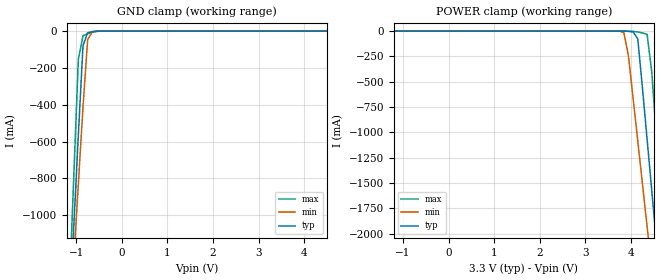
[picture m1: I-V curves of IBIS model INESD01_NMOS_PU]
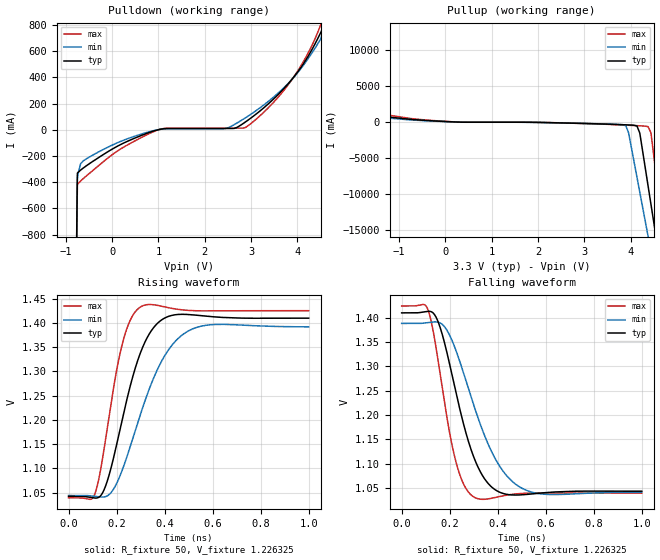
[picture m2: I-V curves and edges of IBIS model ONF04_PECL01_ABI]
|   This file is an IBIS representation of the   |
|   Integrated Device Technology Inc   |
|   ICS844201I-45   |
|   FEMTOCLOCKS CRYSTAL-TO-LVDS CLOCK GENERATOR   |
[IBIS Ver]   4.1
[File name]   844201i_45_3v3.ibs
[File Rev]   1.0
[Date]   3 Mar 2010
[Source]   Originated at Integrated Device Technology, Inc.
[Disclaimer]
IDT hereby grants the user of this IBIS model a non-exclusive,
nontransferable license to use this IBIS model under the following terms.
Before using this IBIS model, the user should read this license.
If the user does not accept these terms,  the IBIS model should be
returned to IDT within 30 days.
   The user is granted this license only to use the IBIS model and
is not granted rights to sell, load, rent, lease or license the IBIS
model in whole or in part, or in modified form to anyone other than
user. User may modify the IBIS model to suit its specific
applications but rights to derivative works and such modifications
shall belong to IDT.
   This IBIS model is provided on an "AS IS" basis and IDT makes
absolutely no warranty with respect to the information contained
herein. IDT DISCLAIMS AND CUSTOMER WAIVES ALL WARRANTIES, EXPRESS
OR IMPLIED, INCLUDING WARRANTIES OF MERCHANTABILITY OR FITNESS FOR
A PARTICULAR PURPOSE. The entire risk as to quality and performance
is with the Customer. ACCORDINGLY, IN NO EVENT SHALL THE COMPANY BE
LIABLE FOR ANY DAMAGES, WHETHER IN CONTRACT OR TORT,INCLUDING ANY
LOST PROFITS OR OTHER INCIDENTAL, CONSEQUENTIAL, EXEMPLARY, OR
PUNITIVE DAMAGES ARISING OUT OF THE USE OR APPLICATION OF THE IBIS
model provided in this package. Further, IDT reserves the right to
make changes without notice to any product herein to improve
reliability, function, or design. IDT does not convey any license
under patent rights or any other intellectual property rights,
including those of third parties.
   IDT is not obligated to provide maintenance or support
for the licensed IBIS model.
[Copyright]   Copyright 2010 by IDT Inc.
[Component]   ICS844201KI-45
[Manufacturer] Integrated Device Technology, Inc.
[Package]
|QFN 16
|lead + wire   typ   min   max
R_pkg   72.4655m   58.886m   86.045m
L_pkg   1.47175nH   1.11650nH   1.77850n
C_pkg   0.07747pF   0.07444pF   0.08050pF
[Pin] signal_name  model_name   R_pin   L_pin   C_pin
1   NC   NC   86.045m   1.77850nH   0.08050pF
2   XTAL_IN   NC   58.886m   1.11650nH   0.07444pF
3   XTAL_OUT  NC   58.886m   1.11650nH   0.07444pF
4   FSEL   INESD01_NMOS_PU   86.045m   1.77850nH   0.08050pF
5   GND   GND   86.045m   1.77850nH   0.08050pF
6   NC   NC   58.886m   1.11650nH   0.07444pF
7   NC   NC   58.886m   1.11650nH   0.07444pF
8   NC   NC   86.045m   1.77850nH   0.08050pF
9   NC   NC   86.045m   1.77850nH   0.08050pF
10   VDD   POWER   58.886m   1.11650nH   0.07444pF
11   nQ   ONF04_PECL01_ABI   58.886m   1.11650nH   0.07444pF
12   Q   ONF04_PECL01_ABI   86.045m   1.77850nH   0.08050pF
13   NC   NC   86.045m   1.77850nH   0.08050pF
14   NC   NC   58.886m   1.11650nH   0.07444pF
15   NC   NC   58.886m   1.11650nH   0.07444pF
16   GND   GND   86.045m   1.77850nH   0.08050pF
[Diff Pin]   inv_pin   vdiff   tdelay_typ   tdelay_min   tdelay_max
12   11   NA   0   0   0
| Models and submodels in the file (2): INESD01_NMOS_PU (Input), ONF04_PECL01_ABI (Output)
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[Model]   INESD01_NMOS_PU
Model_type   Input
Polarity   Non-Inverting
Vinl = 0.7V
Vinh = 1.3V
|   typ   min   max
C_comp   2pF   1.5pF   2.5pF
|   typ   min   max
[Voltage range]  3.3V   3.15V   3.45V
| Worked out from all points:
|   GND clamp passes 1 mA (typ) near -0.56 V on its own axis
[GND_clamp]
|Voltage   I(typ)   I(min)   I(max)
-3.3V     -12.24A    -10.56A    -15.06A
-1.157V   -1.578A    -1.673A    -1.45A
-1.055V   -1.071A    -1.251A    -801.8mA
-952.6mV  -564.4mA   -830.8mA   -154mA
-850.5mV  -79.92mA   -410.9mA   -24.97mA
-748.5mV  -8.956mA   -45.87mA   -14.66mA
-646.4mV  -3.019mA   -2.828mA   -6.626mA
-544.3mV  -652uA     -309.6uA   -1.636mA
6.6V      4.435nA    6.865nA    1.283nA
[POWER_clamp]
|Voltage   I(typ)   I(min)   I(max)
-3.3V     4.435nA    5.64nA     1.609nA
3.64V     -5.052uA   -135.1uA   -13.25nA
3.844V    -652uA     -14.51mA   -32.02uA
3.946V    -3.019mA   -250.2mA   -451.4uA
4.048V    -8.956mA   -669.7mA   -3.083mA
4.151V    -79.92mA   -1.09A     -9.442mA
4.355V    -1.071A    -1.933A    -33.35mA
4.457V    -1.578A    -2.355A    -402.1mA
4.559V    -2.085A    -2.777A    -1.05A
4.661V    -2.593A    -3.199A    -1.698A
4.763V    -3.101A    -3.622A    -2.347A
6.6V      -12.24A    -11.24A    -14.01A
[Model]   ONF04_PECL01_ABI
Model_type   Output
Polarity   Non-Inverting
|   typ   min   max
C_comp   2pF   1.5pF   2.5pF
Vmeas = 1.23V
Rref = 50
Cref = 0
Vref = 1.23V
|   typ   min   max
[Voltage range]   3.3V   3.135V   3.465V
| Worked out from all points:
|   slope of the pulldown table from 0 to 0.495 V, typ, clamps not added: 5.82 ohm
|   slope of the pullup table from 0 to 0.495 V, typ, clamps not added: 4.87 ohm
|   rising waveform, R_fixture 50, V_fixture 1.226325: 20-80 % time 113ps typ, 153ps min, 79.3ps max; typ from 1.04 V to 1.41 V
|   falling waveform, R_fixture 50, V_fixture 1.226325: 20-80 % time 113ps typ, 153ps min, 79.3ps max; typ from 1.41 V to 1.04 V
[Pulldown]
|Voltage   I (typ)   I (min)   I (max)
-3.3V     -100.9A    -86.69A    -124.9A
-1.26V    -16.29A    -16.38A    -16.38A
-750mV    -331.1mA   -374.5mA   -417.1mA
-679.8mV  -307.4mA   -259.5mA   -391mA
-559.3mV  -275.6mA   -222.4mA   -353.1mA
1.007V    1.021mA    1.35mA     391.3uA
2.452V    9.664mA    8.841mA    12.24mA
2.874V    58.41mA    90.16mA    16.3mA
3.777V    341.6mA    344.5mA    332.3mA
4.5V      739.2mA    691.8mA    798.4mA
4.928V    1.103A     1.4A       1.268A
6.6V      11.32A     11.27A     11.63A
[Pullup]
|Voltage   I (typ)   I (min)   I (max)
-3.3V     11.37A     10.32A     13.25A
-2.28V    4.031A     4.242A     3.795A
-1.77V    1.283A     1.288A     1.792A
42.99mV   98.06mA    84.35mA    114.1mA
3.898V    -353.3mA   -492.2mA   -392mA
3.958V    -368.8mA   -1.481A    -410mA
4.199V    -1.494A    -9.723A    -487.6mA
4.38V     -8.923A    -15.91A    -606.7mA
4.44V     -11.4A     -17.97A    -1.468A
4.51V     -14.29A    -20.38A    -5.143A
4.928V    -31.5A     -34.72A    -27.13A
6.6V      -100.8A    -92.33A    -115.9A
[Ramp]
|   typ   min   max
dV/dt_r   0.302/0.176n   0.284/0.236n   0.32/0.124n
dV/dt_f   0.302/0.176n   0.284/0.236n   0.32/0.124n
R_load =   50.0000
[Rising Waveform]
R_fixture = 50
V_fixture   =1.226325   |Vcc_typ
V_fixture_min=1.21646  |Vcc_min
V_fixture_max=1.23202  |Vcc_max
C_fixture = 0.0p
| Time   typ   min   max
0s        1.042V     1.044V     1.039V
110.1ps   1.039V     1.042V     1.048V
156.2ps   1.066V     1.042V     1.166V
219.2ps   1.191V     1.091V     1.347V
254.3ps   1.265V     1.141V     1.402V
293.3ps   1.33V      1.202V     1.43V
376.4ps   1.402V     1.31V      1.435V
434.4ps   1.416V     1.356V     1.429V
499.5ps   1.417V     1.383V     1.426V
1ns       1.41V      1.392V     1.425V
[Falling Waveform]
R_fixture = 50
V_fixture   =1.226325   |Vcc_typ
V_fixture_min=1.21646  |Vcc_min
V_fixture_max=1.23202  |Vcc_max
C_fixture = 0.0p
| Time   typ   min   max
0s        1.41V      1.389V     1.425V
110.1ps   1.414V     1.39V      1.416V
156.2ps   1.386V     1.391V     1.298V
219.2ps   1.262V     1.342V     1.117V
254.3ps   1.188V     1.292V     1.062V
293.3ps   1.123V     1.231V     1.034V
376.4ps   1.051V     1.123V     1.029V
434.4ps   1.037V     1.077V     1.035V
499.5ps   1.036V     1.05V      1.039V
1ns       1.043V     1.041V     1.039V
